PROGRAM p04_IL_klic
VAR
	S0: BOOL;
	S1: BOOL;
	S2: BOOL;
	L0: BOOL;
	L1: BOOL;
	L2: BOOL;
	logicneOperacije: p03_IL_logOperacije;
END_VAR

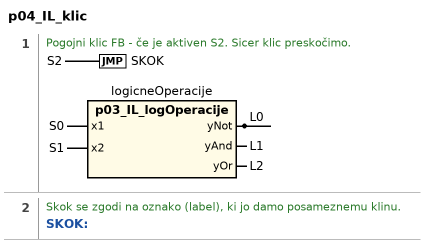
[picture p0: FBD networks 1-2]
// NETWORK 1
// Pogojni klic FB - če je aktiven S2. Sicer klic preskočimo.
IF S2 THEN JMP SKOK; END_IF
logicneOperacije(x1 := S0, x2 := S1, yNot => L0, yAnd => L1, yOr => L2); // p03_IL_logOperacije

// NETWORK 2
// Skok se zgodi na oznako (label), ki jo damo posameznemu klinu.
SKOK:
// instruction list

END_PROGRAM
